(* Logix 5000 AddOnInstructionDefinition export Banner_DFG1_Param_v4; software revision 32.00 *)

TYPE Banner_DFG1_RD_v2 :   // UDT with all of the Read only parameters for DFG1.
STRUCT
   Master_Cycle_Time : INT;
   Min_Cycle_Time : INT;
   M_Sequence_Capability : INT;
   IO_Link_Version_ID : INT;
   Process_Data_Input_Length : INT;
   Process_Data_Output_Length : INT;
   Combined_Vendor_ID : DINT;   // IO-Link Vendor ID
   Vendor_ID1 : INT;
   Vendor_ID2 : INT;
   Combined_Device_ID : DINT;   // IO-Link Device ID
   Device_ID1 : INT;
   Device_ID2 : INT;
   Device_ID3 : INT;
   Serial_Number : STRING;
   Teach_State : SINT;   // 0 =IDLE, 1 = SP1 Success, 4 = Wait for Command, 5 = Busy, 7 = Error
   SP1_TP1 : SINT;   // 0 = Teach point 1 not taught or not successful, 1 = Teach point 1 was successful
   SP1_TP2 : SINT;   // 0 = Teach point 2 not taught or not successful, 1 = Teach point 2 was successful
   SP2_TP1 : SINT;   // 0 = Teach point 2 not taught or not successful, 1 = Teach point 2 was successful
   SP2_TP2 : SINT;   // 0 = Teach point 2 not taught or not successful, 1 = Teach point 2 was successful
   Output_Mode : SINT;   // 0 = Dark Operate, 1 = Light Operate.
   Lower_Hysteresis : DINT;
   Lower_Threshold : DINT;
   Reference : DINT;
   Upper_Hysteresis : DINT;
   Upper_Threshold : DINT;
   Max_Adjustable_Reference : DINT;
   Min_Adjustable_Reference : DINT;
   Max_Teachable_Reference : DINT;
   Min_Teachable_Reference : DINT;
END_STRUCT
END_TYPE

TYPE Banner_DFG1_v2 :   // UDT with all of the parameters needed to work with a Banner DF-G1 IO-Link Sensor.
STRUCT
   Initial_Global_Read : BOOL;   // Determines if all of the IO-Link data has been read into the PLC yet
   Command : INT;   // Value placed in here will activate a read or write to a specifc IO-Link Index
   Read_Data : Banner_DFG1_RD_v2;
   Write_Data : Banner_DFG1_WD_v2;
   Archive_Data : Banner_DFG1_WD_v2;
   Reset : BOOL;   // Resets AOI. This will force a complete parameter read of the sensor.
END_STRUCT
END_TYPE

TYPE Banner_DFG1_WD_v2 :   // UDT with all of the Write only parameters for DFG1.
STRUCT
   System_Command : INT;   // See IODD file for list of commands that can be activated via the System Command interface
   Parameter_Access_Lock : SINT;   // Write access to all read/write parameters is block when this bit is ON.
   Data_Storage_Lock : SINT;   // Data storage mechanism is inhibited when bit is ON.
   Local_Parameterization_Lock : SINT;   // Parameteriation via local control elementes is inhibited.
   Local_User_Interface_Lock : SINT;   // Operation of the hmi on the device is disabled.
   BDC1_Setpoint_SP1 : DINT;   // Switch point value
   BDC1_Setpoint_SP2 : DINT;   // Unused
   BDC1_Swithpoint_Logic : INT;   // 0 = Light Operate, 1 = Dark Operate
   BDC1_BDC_Mode : INT;   // 1 = Single Point, 128 = Window Set, 129 = Light Set, 130 = Dark Set
   BDC1_Hysteresis : DINT;   // User selectable Hysteresis. 0 = 1.0x, 1 = 1.5x, and 2 = 2.5x.
   Off_Delay_On_Oneshot_Time : DINT;   // Delay in ms.
   On_Delay_Off_Oneshot_Time : DINT;   // Delay in ms.
   Delay_Mode : SINT;   // 0 = Off On Delay, 3 = Off Oneshot, 12 = On Oneshot.
   Process_Data_Filter_Update_Time : DINT;   // Value*.1ms. Amount of time to collect average sample for process data.
   Auto_Threshold_Response_Time : INT;   // 14 = 2.5s, 15 = 5s, 16 = 10s, 17 = 20s. Used in Light/Dark/Window Set only.
   Offset_Percent : DINT;   // Offset percent from taught condition in Window, Light or Dark Set modes only.
   Auto_Treshold : SINT;   // 0 = Disabled, 3 = Enabled. Algorithm caontinuously tracks slow changes in taught condition and optimizes thresholds.
   Teach_Selection : INT;   // 0 = 2Pt, 1 = Dynamic, 2 = Window, 3 = Light, 4 = Dark, 5 = Cal.
   Response_Speed : INT;   // 0 = 200, 1 = 500, 2 = 2000, 3 = 5000 microseconds.
   Gain_Mode : SINT;   // 0 = Fixed, 2 = Auto.
   Gain_Level : SINT;   // 0 = Gain 1, 1 = Gain 2, 2 = Gain 3, 3 = Gain 4, 4= Gain 5, 5 = Gain 6, 6 = Gain 7, 7 = Gain 8.
   Display_Orientation : SINT;   // 0 = Normal, 1 = Flipped.
   ECO_Mode : SINT;   // 0 = Disabled, 1 = Enabled.
   Signal_Theshold_Readout : SINT;   // 0 = Numeric, 1 = Percentage.
END_STRUCT
END_TYPE

TYPE Banner_IOL_Port_v4 :   // UDT that has all of the data items necessary to communicate with a specific Port on a IO-Link Master
STRUCT
   Port_Controlled : INT;   // Each bit represents a port on an IO-Link Master. Set to 1 to tell AOI to control that port.
   Port_Activate : INT;   // Each bit represents a port on an IO-Link Master. When ON that port will process any commands in queue.
   Port_Read : INT;   // Each bit represents a port on an IO-Link Master. Used to determine when device AOI has requested a Read command.
   Port_Write : INT;   // Each bit represents a port on an IO-Link Master. Used to determine when device AOI has requested a Write command.
   Port_RW_Complete : INT;   // Each bit represents a port on an IO-Link Master. Tells device AOI that Read or Write request has been completed.
   Port_Device_Read : INT;
   Data_Transfer : SINT[190];   // Array to transfer data from IO-Master to device AOIs.
END_STRUCT
END_TYPE

ADD_ON_INSTRUCTION Banner_DFG1_Param_v4   (* revision 4.0, vendor Banner Engineering *)
// AOI to read and write parameter data to an IO-Link DF-G1.
VAR_IN_OUT
   DFG1 : Banner_DFG1_v2; {required}
   Port_Data : Banner_IOL_Port_v4; {required}
END_VAR
VAR_INPUT
   Port : DINT; {required}
END_VAR
VAR
   Local_Control : DINT; {access None}
   Global_Read_Command_Value : INT; {access None}
   Global_Write_Command_Value : INT; {access None}
   Error_Generated : BOOL; {access None}
   Command_Being_Processed : BOOL; {access None}
   Update_Archive : BOOL; {access None}
   Index_Write_Inprocess : DINT; {access None}
   Index_Write_Control : DINT; {access None}
   Inprocess_Index : DINT; {access None}
END_VAR

ROUTINE Logic   (* ladder *)
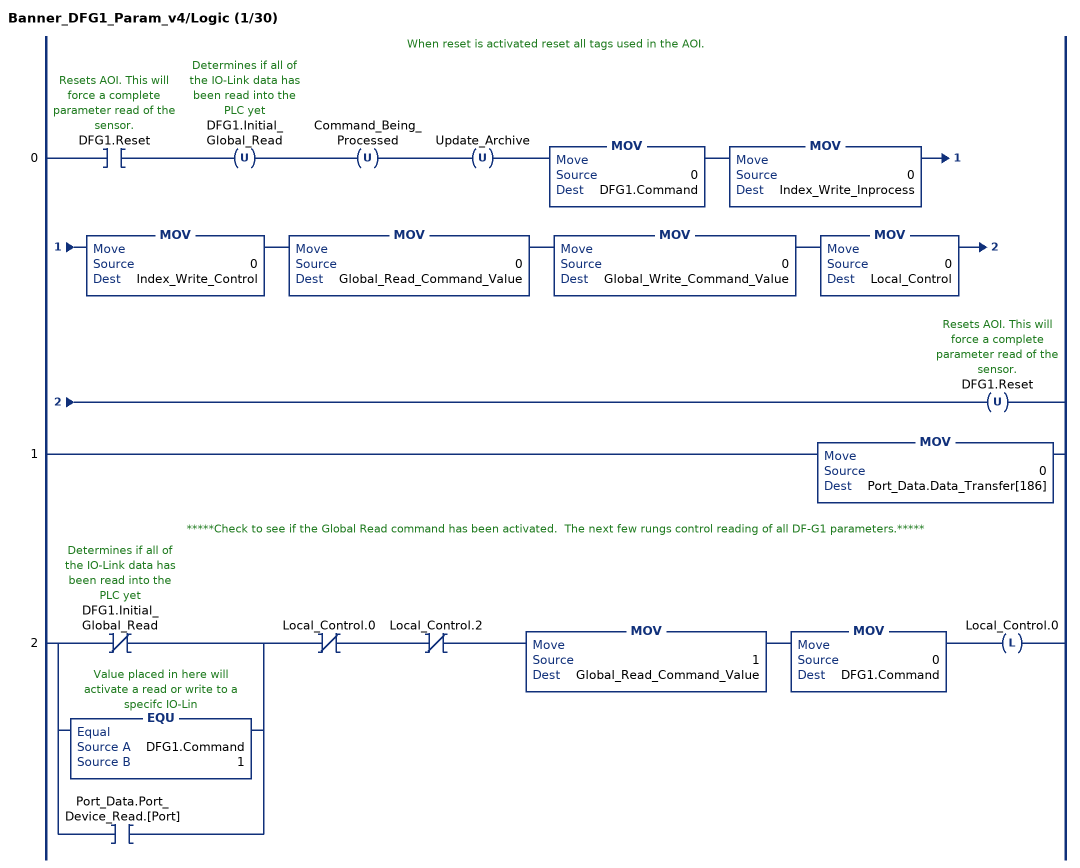
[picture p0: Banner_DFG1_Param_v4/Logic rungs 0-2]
   // When reset is activated reset all tags used in the AOI.
   0: XIC(DFG1.Reset)OTU(DFG1.Initial_Global_Read)OTU(Command_Being_Processed)OTU(Update_Archive)MOV(0,DFG1.Command)MOV(0,Index_Write_Inprocess)MOV(0,Index_Write_Control)MOV(0,Global_Read_Command_Value)MOV(0,Global_Write_Command_Value)MOV(0,Local_Control)OTU(DFG1.Reset);
   1: MOV(0,Port_Data.Data_Transfer[186]);
   // *****Check to see if the Global Read command has been activated.  The next few rungs control reading of all DF-G1 parameters.*****
   2: [XIO(DFG1.Initial_Global_Read) ,EQU(DFG1.Command,1) ,XIC(Port_Data.Port_Device_Read.[Port]) ]XIO(Local_Control.0)XIO(Local_Control.2)MOV(1,Global_Read_Command_Value)MOV(0,DFG1.Command)OTL(Local_Control.0);
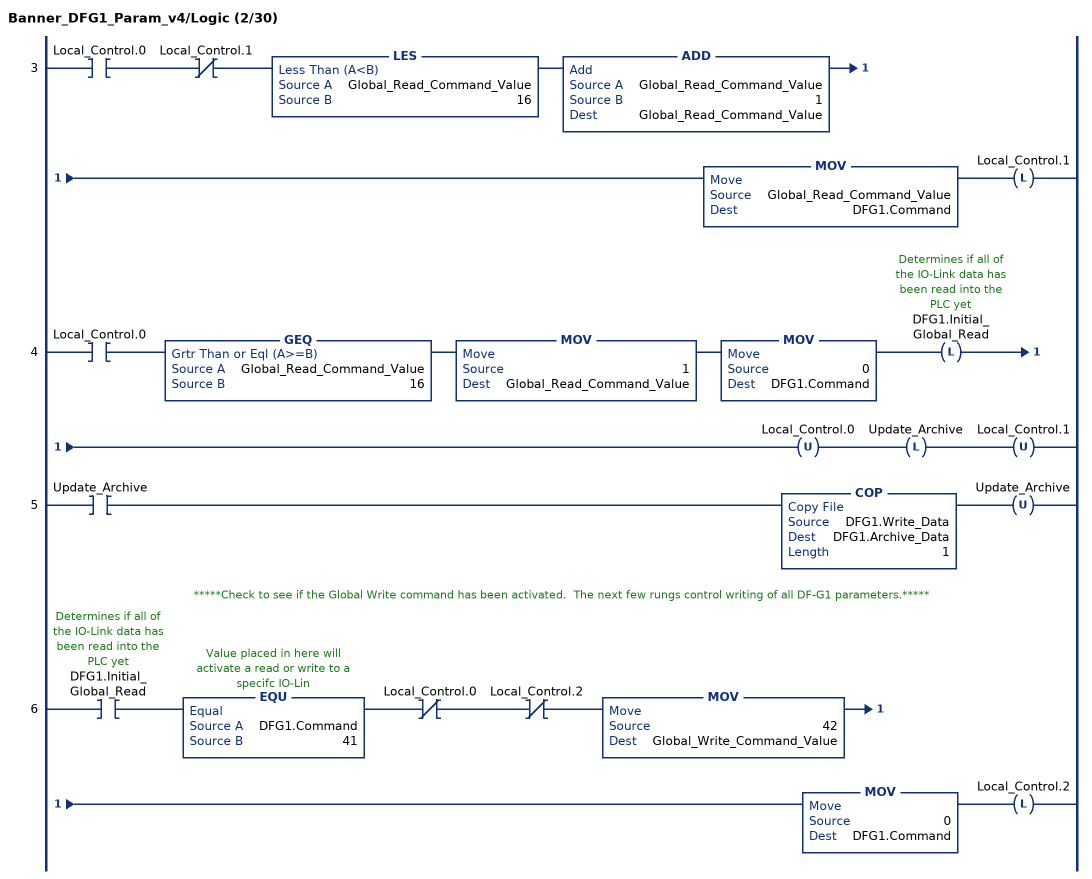
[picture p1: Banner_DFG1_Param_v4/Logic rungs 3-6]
   3: XIC(Local_Control.0)XIO(Local_Control.1)LES(Global_Read_Command_Value,16)ADD(Global_Read_Command_Value,1,Global_Read_Command_Value)MOV(Global_Read_Command_Value,DFG1.Command)OTL(Local_Control.1);
   4: XIC(Local_Control.0)GEQ(Global_Read_Command_Value,16)MOV(1,Global_Read_Command_Value)MOV(0,DFG1.Command)OTL(DFG1.Initial_Global_Read)OTU(Local_Control.0)OTL(Update_Archive)OTU(Local_Control.1);
   5: XIC(Update_Archive)COP(DFG1.Write_Data,DFG1.Archive_Data,1)OTU(Update_Archive);
   // *****Check to see if the Global Write command has been activated.  The next few rungs control writing of all DF-G1 parameters.*****
   6: XIC(DFG1.Initial_Global_Read)EQU(DFG1.Command,41)XIO(Local_Control.0)XIO(Local_Control.2)MOV(42,Global_Write_Command_Value)MOV(0,DFG1.Command)OTL(Local_Control.2);
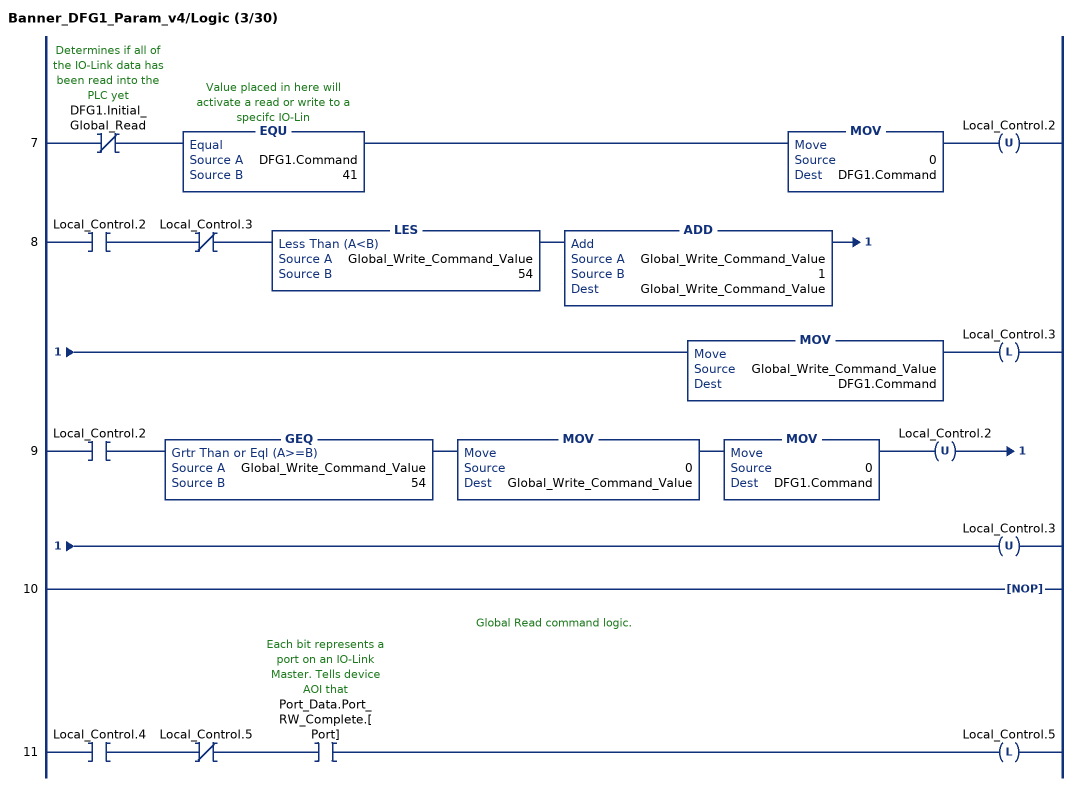
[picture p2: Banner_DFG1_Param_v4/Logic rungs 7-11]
   7: XIO(DFG1.Initial_Global_Read)EQU(DFG1.Command,41)MOV(0,DFG1.Command)OTU(Local_Control.2);
   8: XIC(Local_Control.2)XIO(Local_Control.3)LES(Global_Write_Command_Value,54)ADD(Global_Write_Command_Value,1,Global_Write_Command_Value)MOV(Global_Write_Command_Value,DFG1.Command)OTL(Local_Control.3);
   9: XIC(Local_Control.2)GEQ(Global_Write_Command_Value,54)MOV(0,Global_Write_Command_Value)MOV(0,DFG1.Command)OTU(Local_Control.2)OTU(Local_Control.3);
   10: NOP();
   // Global Read command logic.
   11: XIC(Local_Control.4)XIO(Local_Control.5)XIC(Port_Data.Port_RW_Complete.[Port])OTL(Local_Control.5);
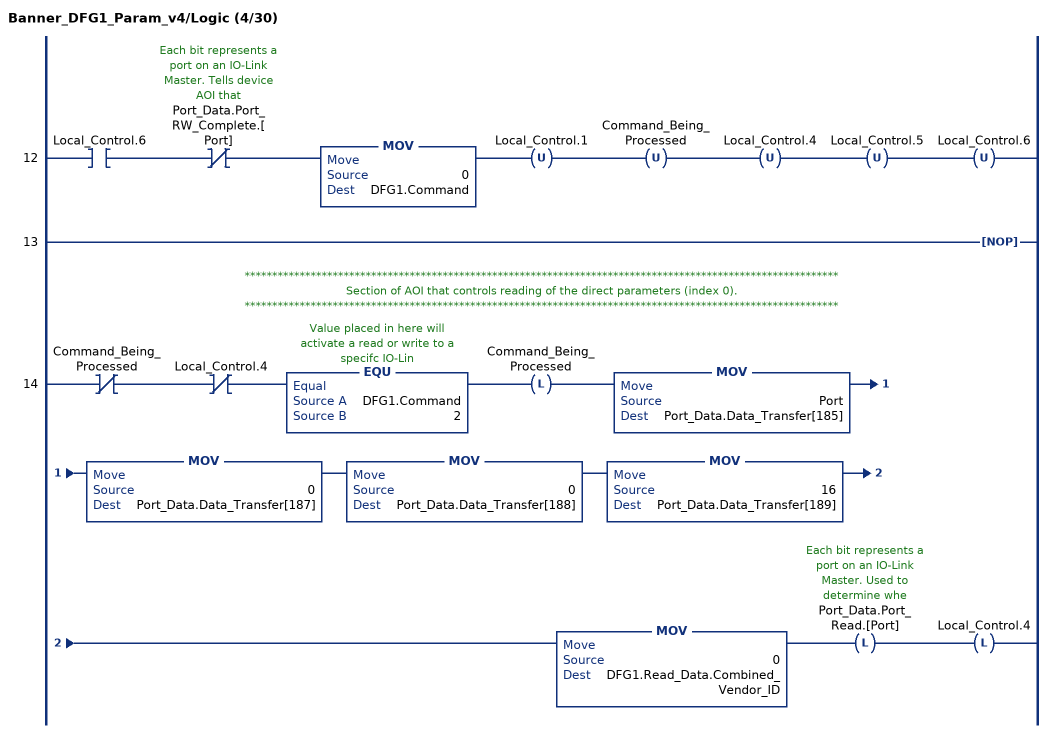
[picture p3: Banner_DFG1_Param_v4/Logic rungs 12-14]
   12: XIC(Local_Control.6)XIO(Port_Data.Port_RW_Complete.[Port])MOV(0,DFG1.Command)OTU(Local_Control.1)OTU(Command_Being_Processed)OTU(Local_Control.4)OTU(Local_Control.5)OTU(Local_Control.6);
   13: NOP();
   // ************************************************************************************************************
   // Section of AOI that controls reading of the direct parameters (index 0).
   // ************************************************************************************************************
   14: XIO(Command_Being_Processed)XIO(Local_Control.4)EQU(DFG1.Command,2)OTL(Command_Being_Processed)MOV(Port,Port_Data.Data_Transfer[185])MOV(0,Port_Data.Data_Transfer[187])MOV(0,Port_Data.Data_Transfer[188])MOV(16,Port_Data.Data_Transfer[189])MOV(0,DFG1.Read_Data.Combined_Vendor_ID)OTL(Port_Data.Port_Read.[Port])OTL(Local_Control.4);
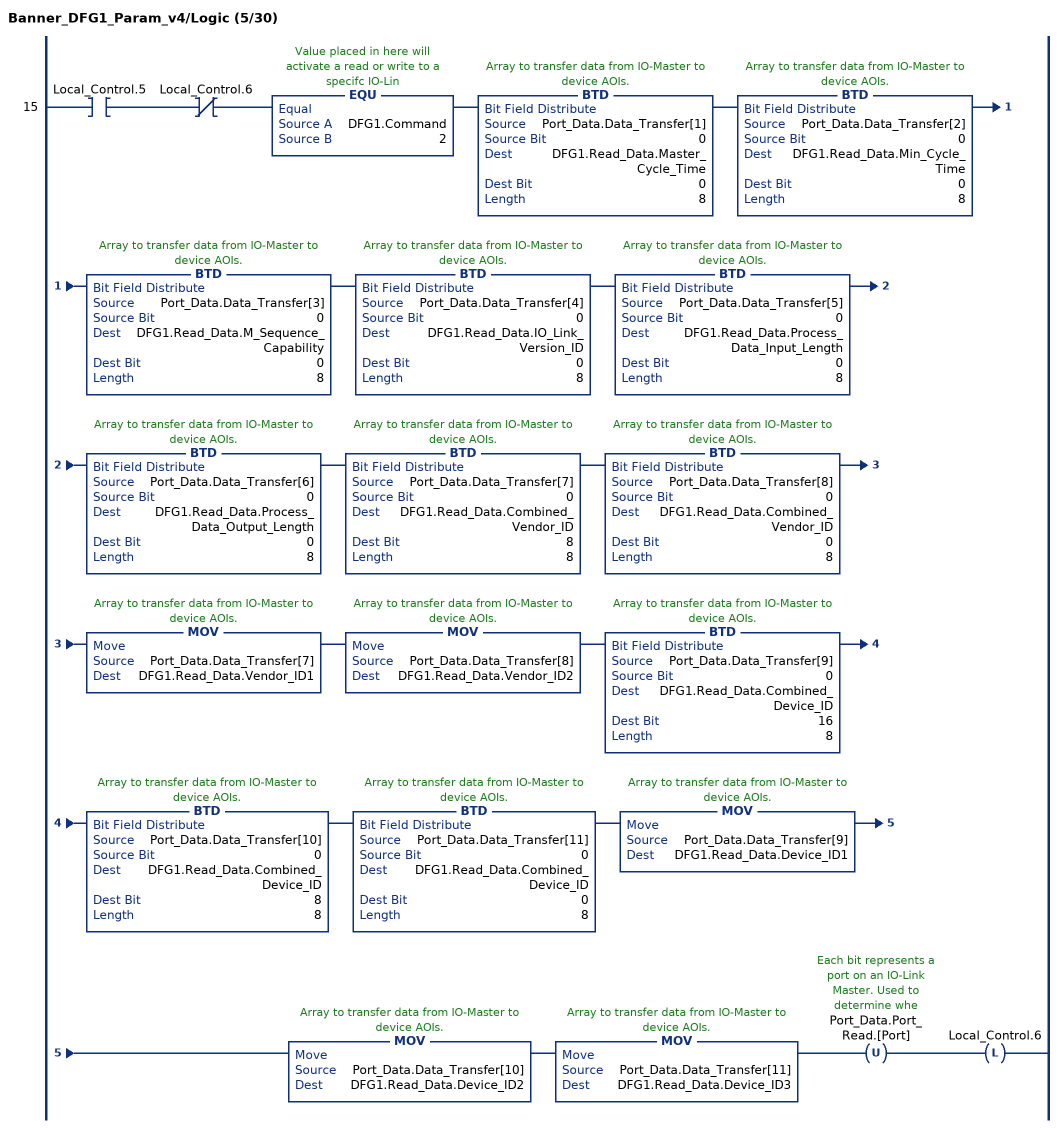
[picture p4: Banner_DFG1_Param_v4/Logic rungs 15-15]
   15: XIC(Local_Control.5)XIO(Local_Control.6)EQU(DFG1.Command,2)BTD(Port_Data.Data_Transfer[1],0,DFG1.Read_Data.Master_Cycle_Time,0,8)BTD(Port_Data.Data_Transfer[2],0,DFG1.Read_Data.Min_Cycle_Time,0,8)BTD(Port_Data.Data_Transfer[3],0,DFG1.Read_Data.M_Sequence_Capability,0,8)BTD(Port_Data.Data_Transfer[4],0,DFG1.Read_Data.IO_Link_Version_ID,0,8)BTD(Port_Data.Data_Transfer[5],0,DFG1.Read_Data.Process_Data_Input_Length,0,8)BTD(Port_Data.Data_Transfer[6],0,DFG1.Read_Data.Process_Data_Output_Length,0,8)BTD(Port_Data.Data_Transfer[7],0,DFG1.Read_Data.Combined_Vendor_ID,8,8)BTD(Port_Data.Data_Transfer[8],0,DFG1.Read_Data.Combined_Vendor_ID,0,8)MOV(Port_Data.Data_Transfer[7],DFG1.Read_Data.Vendor_ID1)MOV(Port_Data.Data_Transfer[8],DFG1.Read_Data.Vendor_ID2)BTD(Port_Data.Data_Transfer[9],0,DFG1.Read_Data.Combined_Device_ID,16,8)BTD(Port_Data.Data_Transfer[10],0,DFG1.Read_Data.Combined_Device_ID,8,8)BTD(Port_Data.Data_Transfer[11],0,DFG1.Read_Data.Combined_Device_ID,0,8)MOV(Port_Data.Data_Transfer[9],DFG1.Read_Data.Device_ID1)MOV(Port_Data.Data_Transfer[10],DFG1.Read_Data.Device_ID2)MOV(Port_Data.Data_Transfer[11],DFG1.Read_Data.Device_ID3)OTU(Port_Data.Port_Read.[Port])OTL(Local_Control.6);
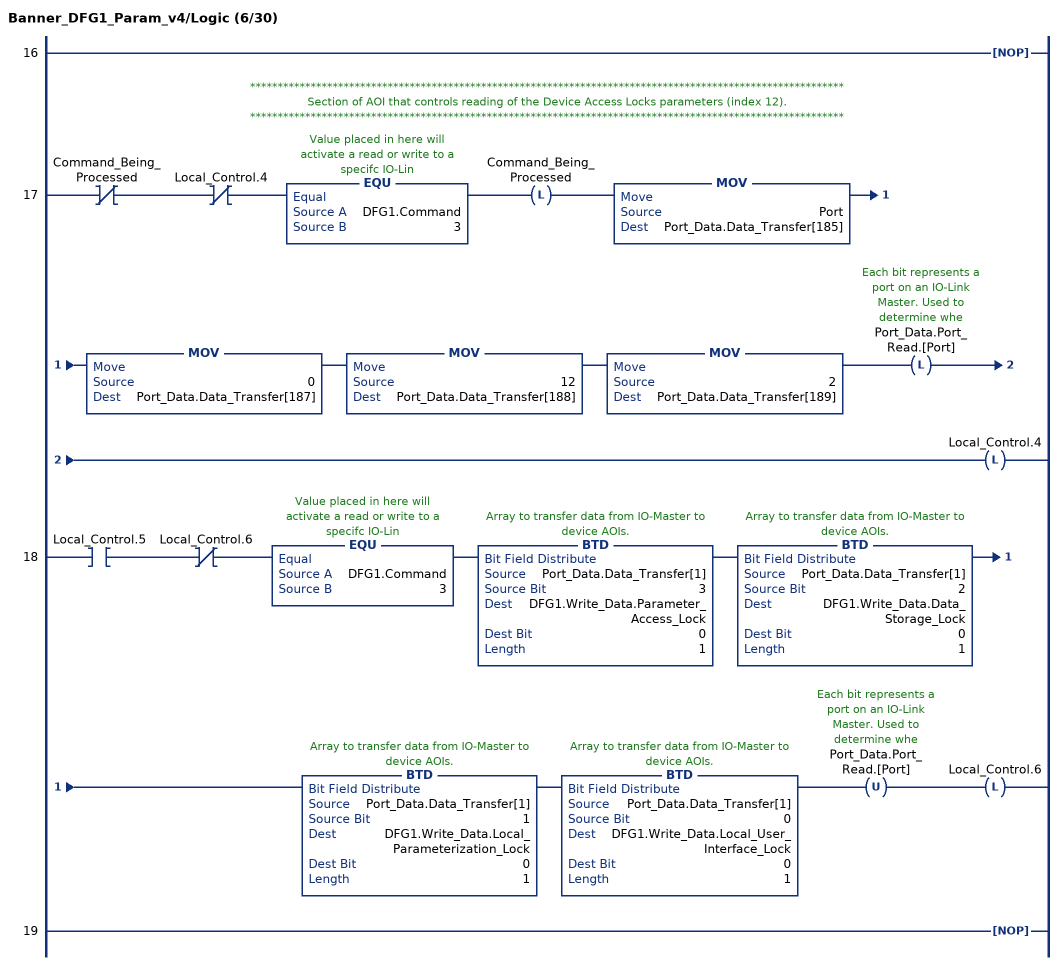
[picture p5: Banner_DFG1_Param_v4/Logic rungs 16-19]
   16: NOP();
   // ************************************************************************************************************
   // Section of AOI that controls reading of the Device Access Locks parameters (index 12).
   // ************************************************************************************************************
   17: XIO(Command_Being_Processed)XIO(Local_Control.4)EQU(DFG1.Command,3)OTL(Command_Being_Processed)MOV(Port,Port_Data.Data_Transfer[185])MOV(0,Port_Data.Data_Transfer[187])MOV(12,Port_Data.Data_Transfer[188])MOV(2,Port_Data.Data_Transfer[189])OTL(Port_Data.Port_Read.[Port])OTL(Local_Control.4);
   18: XIC(Local_Control.5)XIO(Local_Control.6)EQU(DFG1.Command,3)BTD(Port_Data.Data_Transfer[1],3,DFG1.Write_Data.Parameter_Access_Lock,0,1)BTD(Port_Data.Data_Transfer[1],2,DFG1.Write_Data.Data_Storage_Lock,0,1)BTD(Port_Data.Data_Transfer[1],1,DFG1.Write_Data.Local_Parameterization_Lock,0,1)BTD(Port_Data.Data_Transfer[1],0,DFG1.Write_Data.Local_User_Interface_Lock,0,1)OTU(Port_Data.Port_Read.[Port])OTL(Local_Control.6);
   19: NOP();
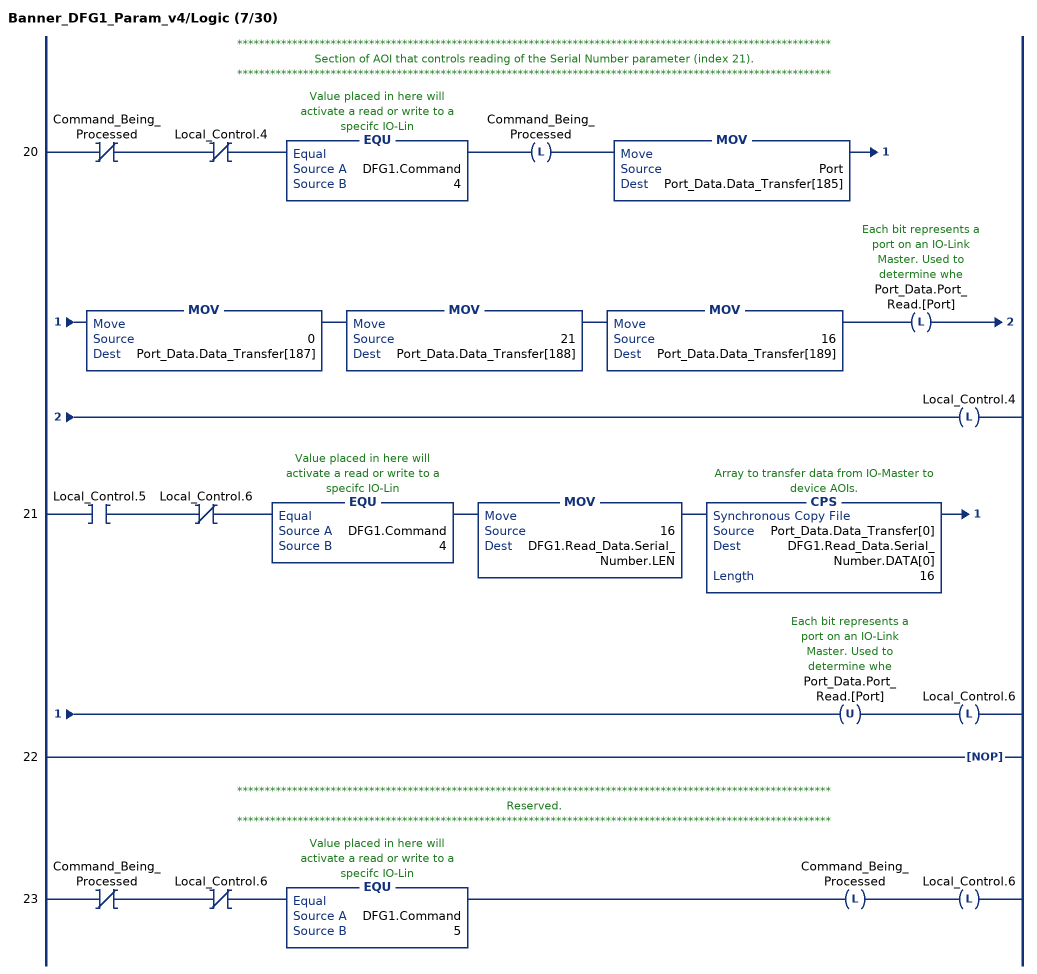
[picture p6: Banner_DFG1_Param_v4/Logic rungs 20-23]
   // ************************************************************************************************************
   // Section of AOI that controls reading of the Serial Number parameter (index 21).
   // ************************************************************************************************************
   20: XIO(Command_Being_Processed)XIO(Local_Control.4)EQU(DFG1.Command,4)OTL(Command_Being_Processed)MOV(Port,Port_Data.Data_Transfer[185])MOV(0,Port_Data.Data_Transfer[187])MOV(21,Port_Data.Data_Transfer[188])MOV(16,Port_Data.Data_Transfer[189])OTL(Port_Data.Port_Read.[Port])OTL(Local_Control.4);
   21: XIC(Local_Control.5)XIO(Local_Control.6)EQU(DFG1.Command,4)MOV(16,DFG1.Read_Data.Serial_Number.LEN)CPS(Port_Data.Data_Transfer[0],DFG1.Read_Data.Serial_Number.DATA[0],16)OTU(Port_Data.Port_Read.[Port])OTL(Local_Control.6);
   22: NOP();
   // ************************************************************************************************************
   // Reserved.
   // ************************************************************************************************************
   23: XIO(Command_Being_Processed)XIO(Local_Control.6)EQU(DFG1.Command,5)OTL(Command_Being_Processed)OTL(Local_Control.6);
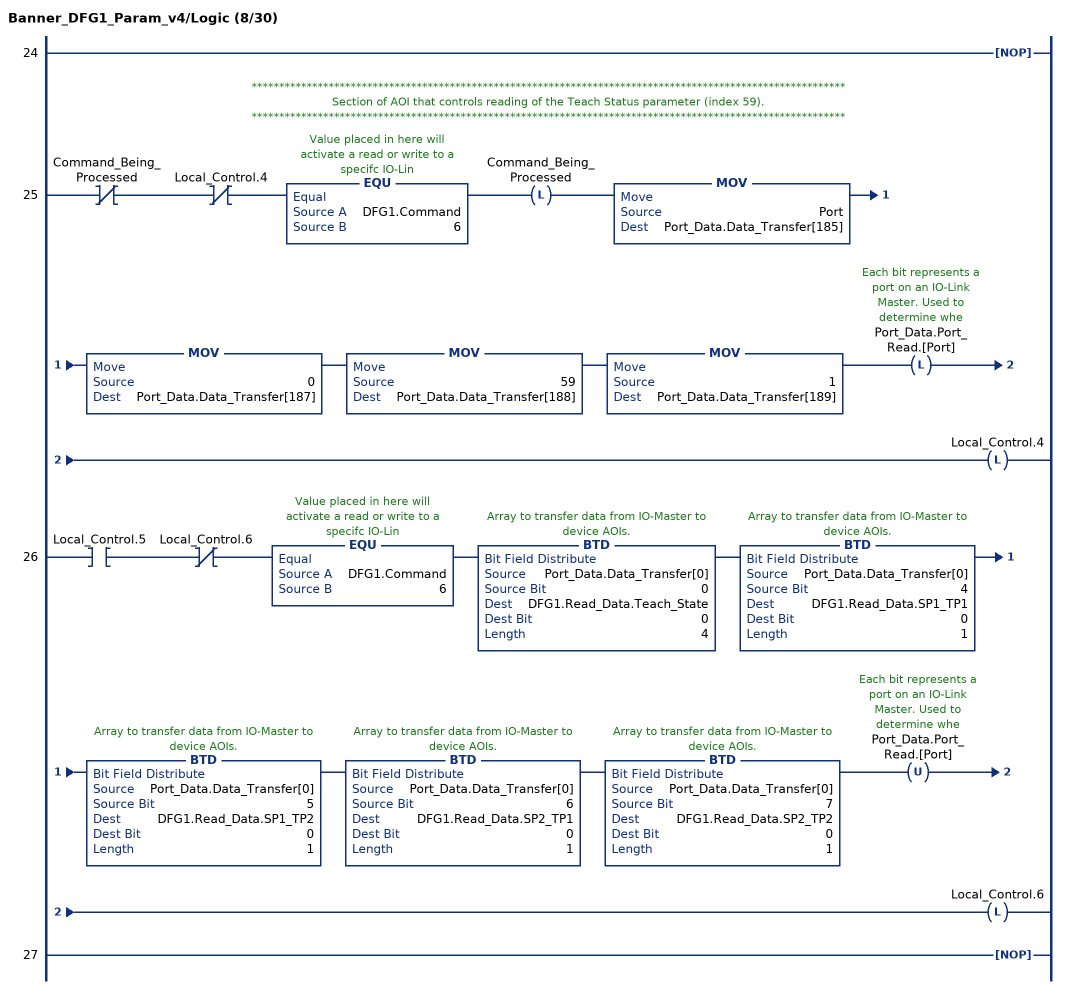
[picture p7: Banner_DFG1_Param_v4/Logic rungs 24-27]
   24: NOP();
   // ************************************************************************************************************
   // Section of AOI that controls reading of the Teach Status parameter (index 59).
   // ************************************************************************************************************
   25: XIO(Command_Being_Processed)XIO(Local_Control.4)EQU(DFG1.Command,6)OTL(Command_Being_Processed)MOV(Port,Port_Data.Data_Transfer[185])MOV(0,Port_Data.Data_Transfer[187])MOV(59,Port_Data.Data_Transfer[188])MOV(1,Port_Data.Data_Transfer[189])OTL(Port_Data.Port_Read.[Port])OTL(Local_Control.4);
   26: XIC(Local_Control.5)XIO(Local_Control.6)EQU(DFG1.Command,6)BTD(Port_Data.Data_Transfer[0],0,DFG1.Read_Data.Teach_State,0,4)BTD(Port_Data.Data_Transfer[0],4,DFG1.Read_Data.SP1_TP1,0,1)BTD(Port_Data.Data_Transfer[0],5,DFG1.Read_Data.SP1_TP2,0,1)BTD(Port_Data.Data_Transfer[0],6,DFG1.Read_Data.SP2_TP1,0,1)BTD(Port_Data.Data_Transfer[0],7,DFG1.Read_Data.SP2_TP2,0,1)OTU(Port_Data.Port_Read.[Port])OTL(Local_Control.6);
   27: NOP();
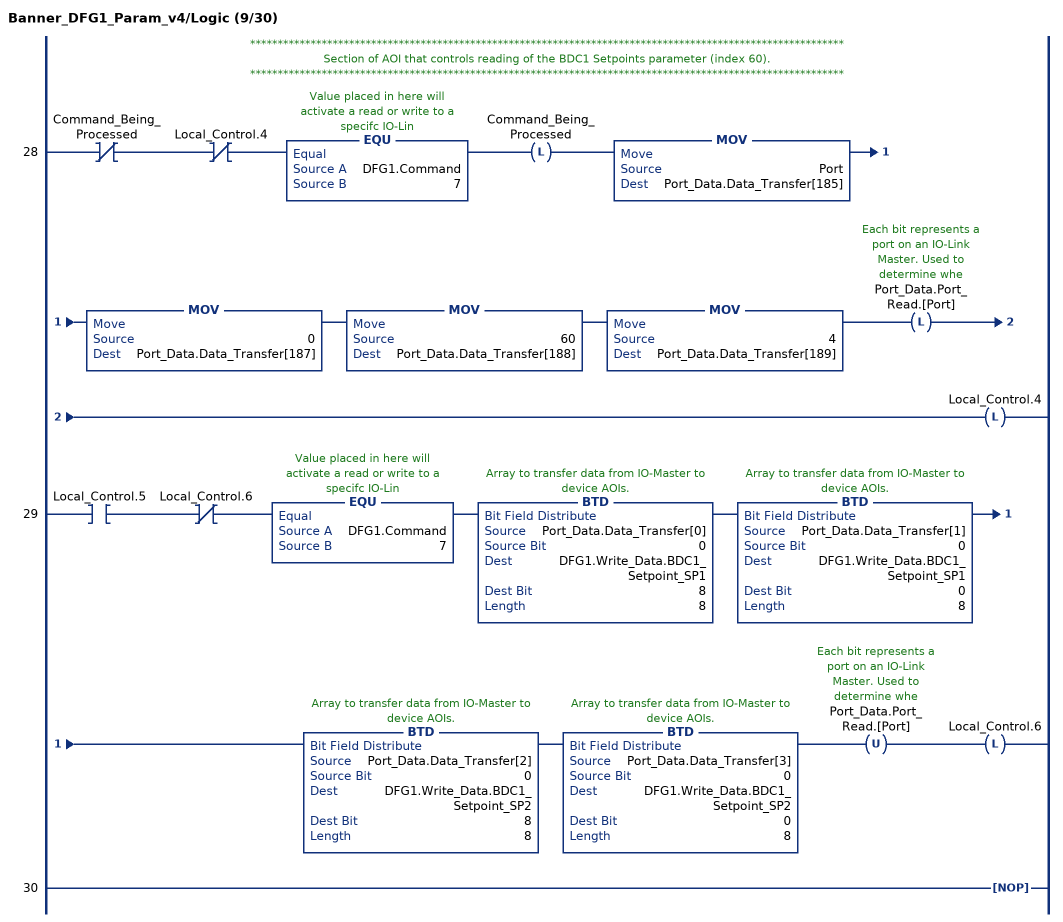
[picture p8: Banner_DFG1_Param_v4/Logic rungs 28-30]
   // ************************************************************************************************************
   // Section of AOI that controls reading of the BDC1 Setpoints parameter (index 60).
   // ************************************************************************************************************
   28: XIO(Command_Being_Processed)XIO(Local_Control.4)EQU(DFG1.Command,7)OTL(Command_Being_Processed)MOV(Port,Port_Data.Data_Transfer[185])MOV(0,Port_Data.Data_Transfer[187])MOV(60,Port_Data.Data_Transfer[188])MOV(4,Port_Data.Data_Transfer[189])OTL(Port_Data.Port_Read.[Port])OTL(Local_Control.4);
   29: XIC(Local_Control.5)XIO(Local_Control.6)EQU(DFG1.Command,7)BTD(Port_Data.Data_Transfer[0],0,DFG1.Write_Data.BDC1_Setpoint_SP1,8,8)BTD(Port_Data.Data_Transfer[1],0,DFG1.Write_Data.BDC1_Setpoint_SP1,0,8)BTD(Port_Data.Data_Transfer[2],0,DFG1.Write_Data.BDC1_Setpoint_SP2,8,8)BTD(Port_Data.Data_Transfer[3],0,DFG1.Write_Data.BDC1_Setpoint_SP2,0,8)OTU(Port_Data.Port_Read.[Port])OTL(Local_Control.6);
   30: NOP();
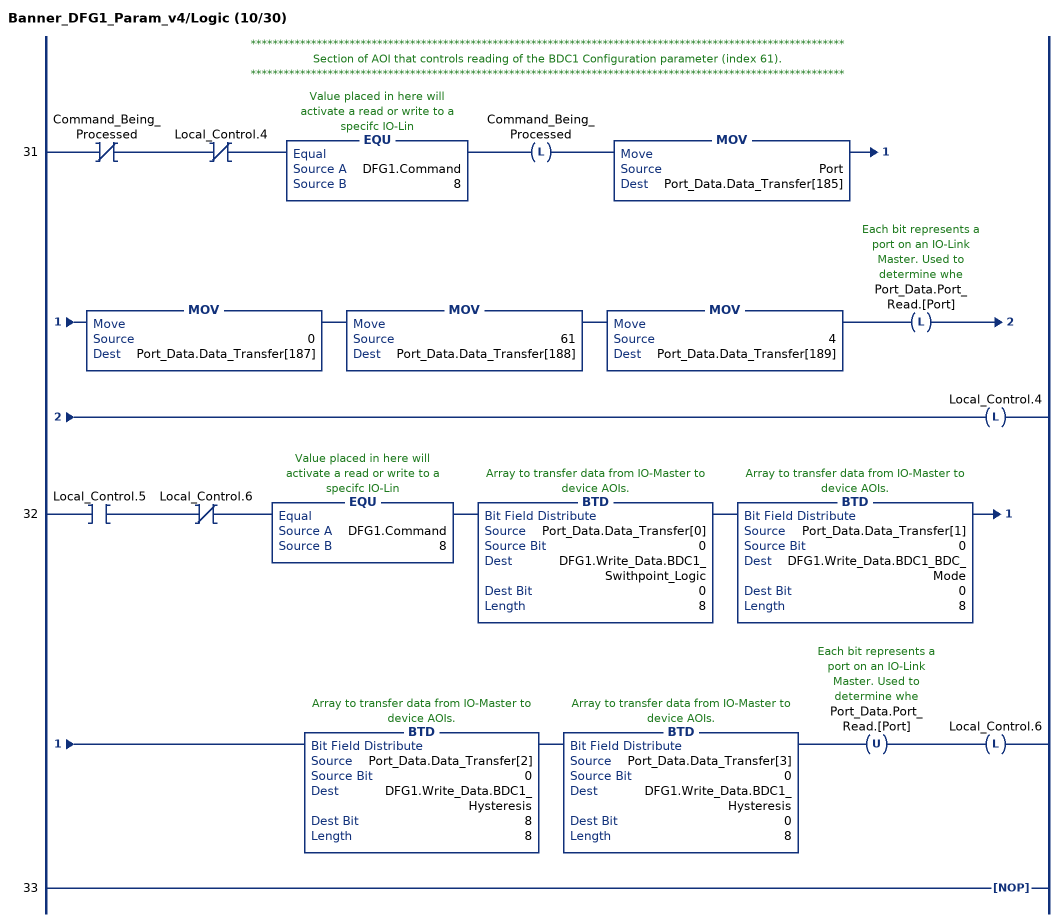
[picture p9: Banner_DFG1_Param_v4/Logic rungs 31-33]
   // ************************************************************************************************************
   // Section of AOI that controls reading of the BDC1 Configuration parameter (index 61).
   // ************************************************************************************************************
   31: XIO(Command_Being_Processed)XIO(Local_Control.4)EQU(DFG1.Command,8)OTL(Command_Being_Processed)MOV(Port,Port_Data.Data_Transfer[185])MOV(0,Port_Data.Data_Transfer[187])MOV(61,Port_Data.Data_Transfer[188])MOV(4,Port_Data.Data_Transfer[189])OTL(Port_Data.Port_Read.[Port])OTL(Local_Control.4);
   32: XIC(Local_Control.5)XIO(Local_Control.6)EQU(DFG1.Command,8)BTD(Port_Data.Data_Transfer[0],0,DFG1.Write_Data.BDC1_Swithpoint_Logic,0,8)BTD(Port_Data.Data_Transfer[1],0,DFG1.Write_Data.BDC1_BDC_Mode,0,8)BTD(Port_Data.Data_Transfer[2],0,DFG1.Write_Data.BDC1_Hysteresis,8,8)BTD(Port_Data.Data_Transfer[3],0,DFG1.Write_Data.BDC1_Hysteresis,0,8)OTU(Port_Data.Port_Read.[Port])OTL(Local_Control.6);
   33: NOP();
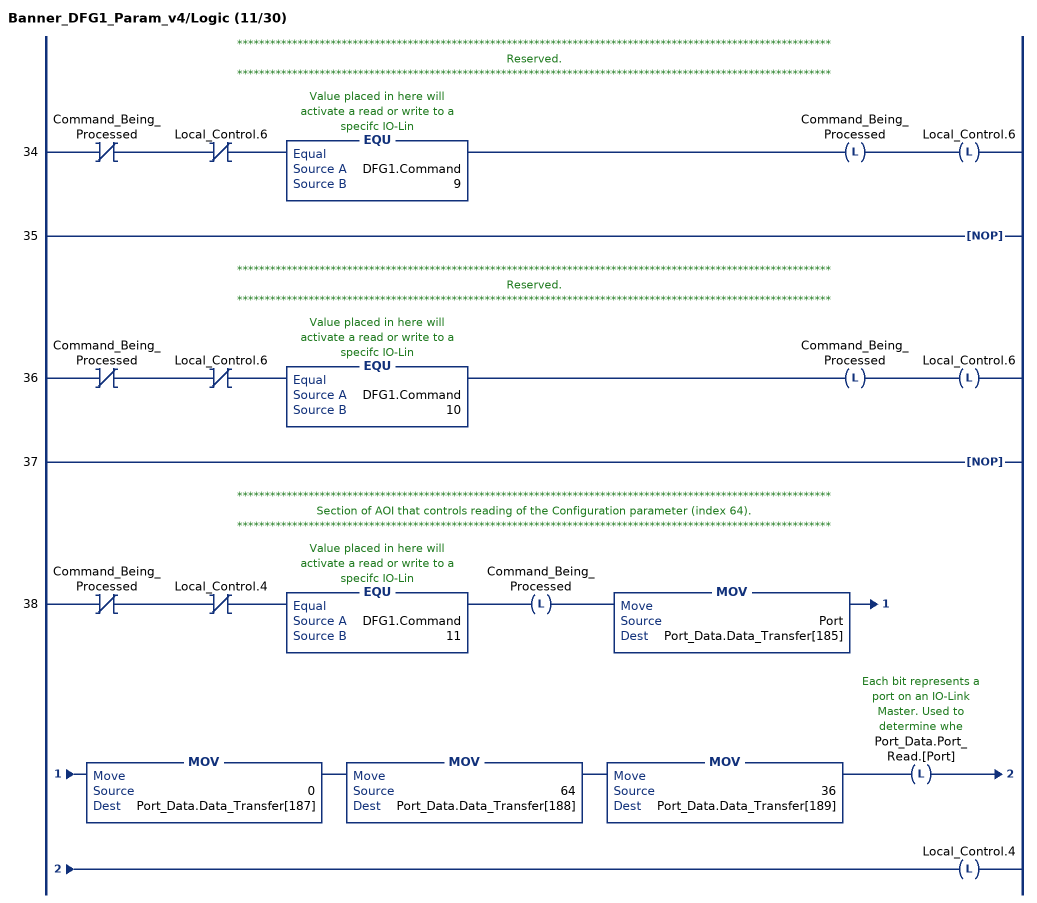
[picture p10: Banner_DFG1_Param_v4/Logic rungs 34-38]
   // ************************************************************************************************************
   // Reserved.
   // ************************************************************************************************************
   34: XIO(Command_Being_Processed)XIO(Local_Control.6)EQU(DFG1.Command,9)OTL(Command_Being_Processed)OTL(Local_Control.6);
   35: NOP();
   // ************************************************************************************************************
   // Reserved.
   // ************************************************************************************************************
   36: XIO(Command_Being_Processed)XIO(Local_Control.6)EQU(DFG1.Command,10)OTL(Command_Being_Processed)OTL(Local_Control.6);
   37: NOP();
   // ************************************************************************************************************
   // Section of AOI that controls reading of the Configuration parameter (index 64).
   // ************************************************************************************************************
   38: XIO(Command_Being_Processed)XIO(Local_Control.4)EQU(DFG1.Command,11)OTL(Command_Being_Processed)MOV(Port,Port_Data.Data_Transfer[185])MOV(0,Port_Data.Data_Transfer[187])MOV(64,Port_Data.Data_Transfer[188])MOV(36,Port_Data.Data_Transfer[189])OTL(Port_Data.Port_Read.[Port])OTL(Local_Control.4);
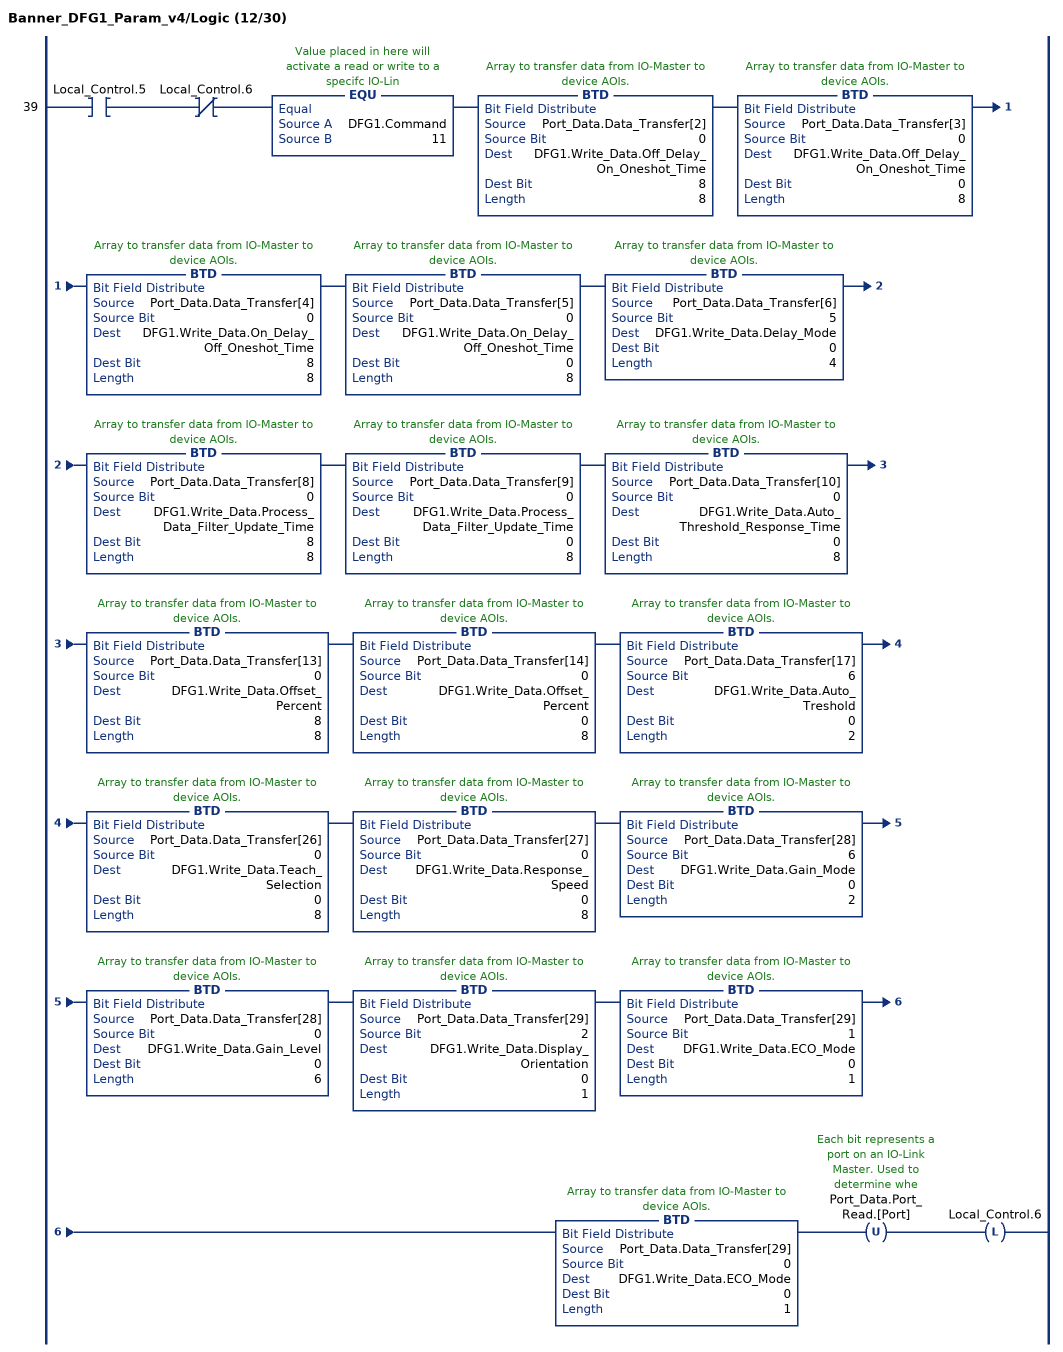
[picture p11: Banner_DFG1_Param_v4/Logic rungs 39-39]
   39: XIC(Local_Control.5)XIO(Local_Control.6)EQU(DFG1.Command,11)BTD(Port_Data.Data_Transfer[2],0,DFG1.Write_Data.Off_Delay_On_Oneshot_Time,8,8)BTD(Port_Data.Data_Transfer[3],0,DFG1.Write_Data.Off_Delay_On_Oneshot_Time,0,8)BTD(Port_Data.Data_Transfer[4],0,DFG1.Write_Data.On_Delay_Off_Oneshot_Time,8,8)BTD(Port_Data.Data_Transfer[5],0,DFG1.Write_Data.On_Delay_Off_Oneshot_Time,0,8)BTD(Port_Data.Data_Transfer[6],5,DFG1.Write_Data.Delay_Mode,0,4)BTD(Port_Data.Data_Transfer[8],0,DFG1.Write_Data.Process_Data_Filter_Update_Time,8,8)BTD(Port_Data.Data_Transfer[9],0,DFG1.Write_Data.Process_Data_Filter_Update_Time,0,8)BTD(Port_Data.Data_Transfer[10],0,DFG1.Write_Data.Auto_Threshold_Response_Time,0,8)BTD(Port_Data.Data_Transfer[13],0,DFG1.Write_Data.Offset_Percent,8,8)BTD(Port_Data.Data_Transfer[14],0,DFG1.Write_Data.Offset_Percent,0,8)BTD(Port_Data.Data_Transfer[17],6,DFG1.Write_Data.Auto_Treshold,0,2)BTD(Port_Data.Data_Transfer[26],0,DFG1.Write_Data.Teach_Selection,0,8)BTD(Port_Data.Data_Transfer[27],0,DFG1.Write_Data.Response_Speed,0,8)BTD(Port_Data.Data_Transfer[28],6,DFG1.Write_Data.Gain_Mode,0,2)BTD(Port_Data.Data_Transfer[28],0,DFG1.Write_Data.Gain_Level,0,6)BTD(Port_Data.Data_Transfer[29],2,DFG1.Write_Data.Display_Orientation,0,1)BTD(Port_Data.Data_Transfer[29],1,DFG1.Write_Data.ECO_Mode,0,1)BTD(Port_Data.Data_Transfer[29],0,DFG1.Write_Data.ECO_Mode,0,1)OTU(Port_Data.Port_Read.[Port])OTL(Local_Control.6);
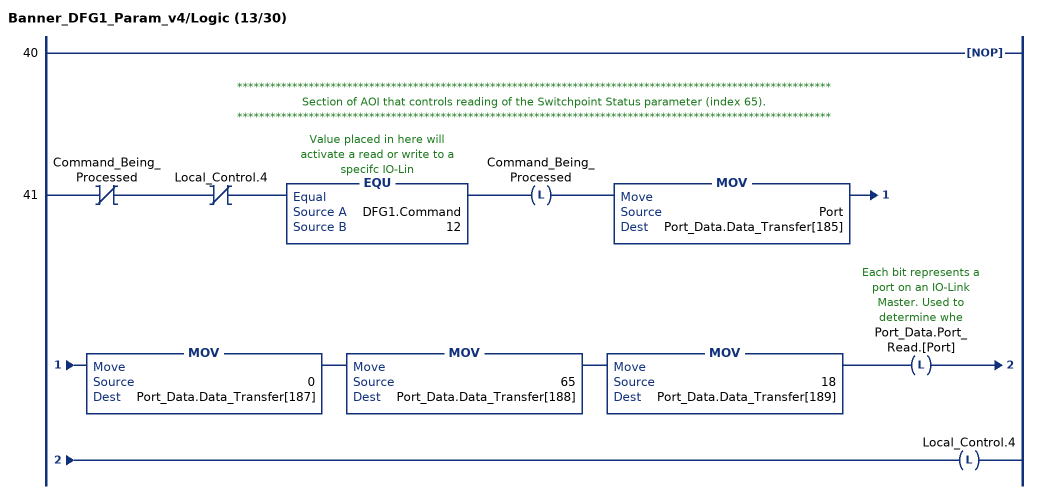
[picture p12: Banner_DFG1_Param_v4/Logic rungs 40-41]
   40: NOP();
   // ************************************************************************************************************
   // Section of AOI that controls reading of the Switchpoint Status parameter (index 65).
   // ************************************************************************************************************
   41: XIO(Command_Being_Processed)XIO(Local_Control.4)EQU(DFG1.Command,12)OTL(Command_Being_Processed)MOV(Port,Port_Data.Data_Transfer[185])MOV(0,Port_Data.Data_Transfer[187])MOV(65,Port_Data.Data_Transfer[188])MOV(18,Port_Data.Data_Transfer[189])OTL(Port_Data.Port_Read.[Port])OTL(Local_Control.4);
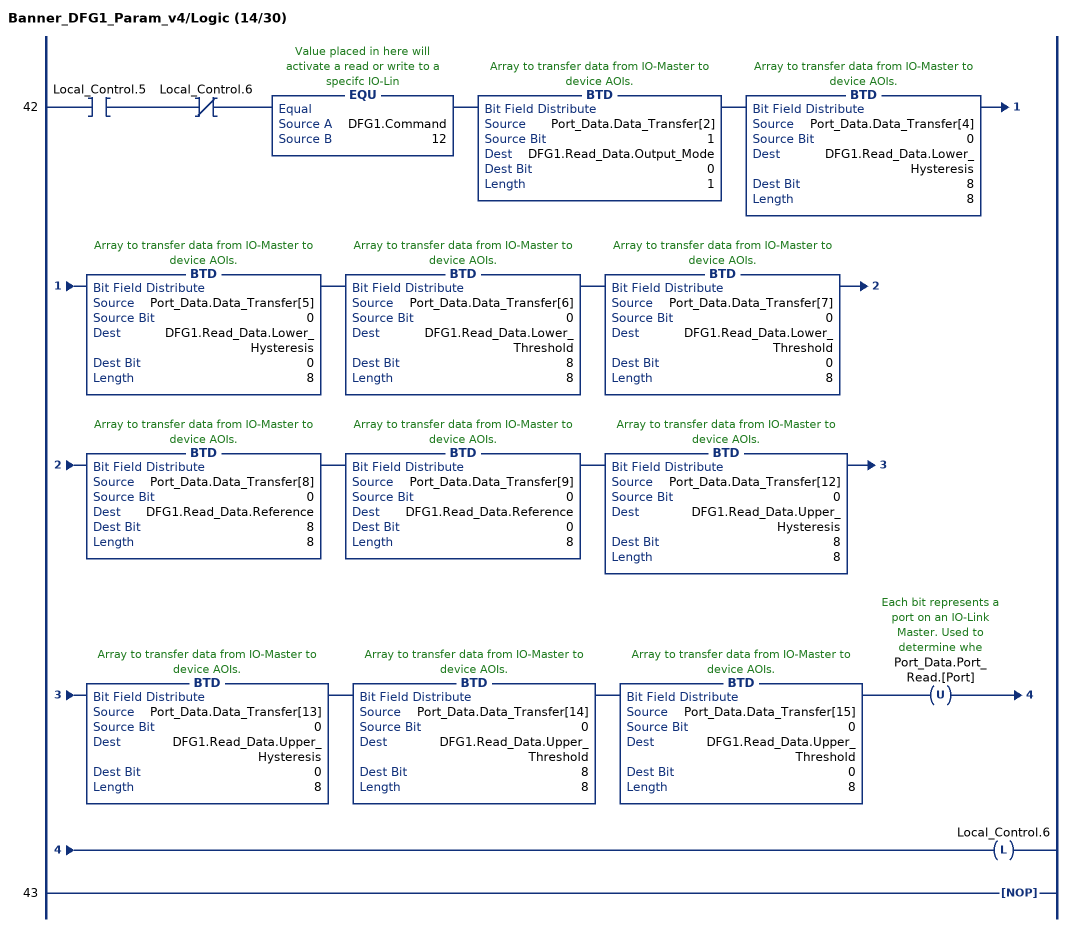
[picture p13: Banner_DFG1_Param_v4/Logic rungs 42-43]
   42: XIC(Local_Control.5)XIO(Local_Control.6)EQU(DFG1.Command,12)BTD(Port_Data.Data_Transfer[2],1,DFG1.Read_Data.Output_Mode,0,1)BTD(Port_Data.Data_Transfer[4],0,DFG1.Read_Data.Lower_Hysteresis,8,8)BTD(Port_Data.Data_Transfer[5],0,DFG1.Read_Data.Lower_Hysteresis,0,8)BTD(Port_Data.Data_Transfer[6],0,DFG1.Read_Data.Lower_Threshold,8,8)BTD(Port_Data.Data_Transfer[7],0,DFG1.Read_Data.Lower_Threshold,0,8)BTD(Port_Data.Data_Transfer[8],0,DFG1.Read_Data.Reference,8,8)BTD(Port_Data.Data_Transfer[9],0,DFG1.Read_Data.Reference,0,8)BTD(Port_Data.Data_Transfer[12],0,DFG1.Read_Data.Upper_Hysteresis,8,8)BTD(Port_Data.Data_Transfer[13],0,DFG1.Read_Data.Upper_Hysteresis,0,8)BTD(Port_Data.Data_Transfer[14],0,DFG1.Read_Data.Upper_Threshold,8,8)BTD(Port_Data.Data_Transfer[15],0,DFG1.Read_Data.Upper_Threshold,0,8)OTU(Port_Data.Port_Read.[Port])OTL(Local_Control.6);
   43: NOP();
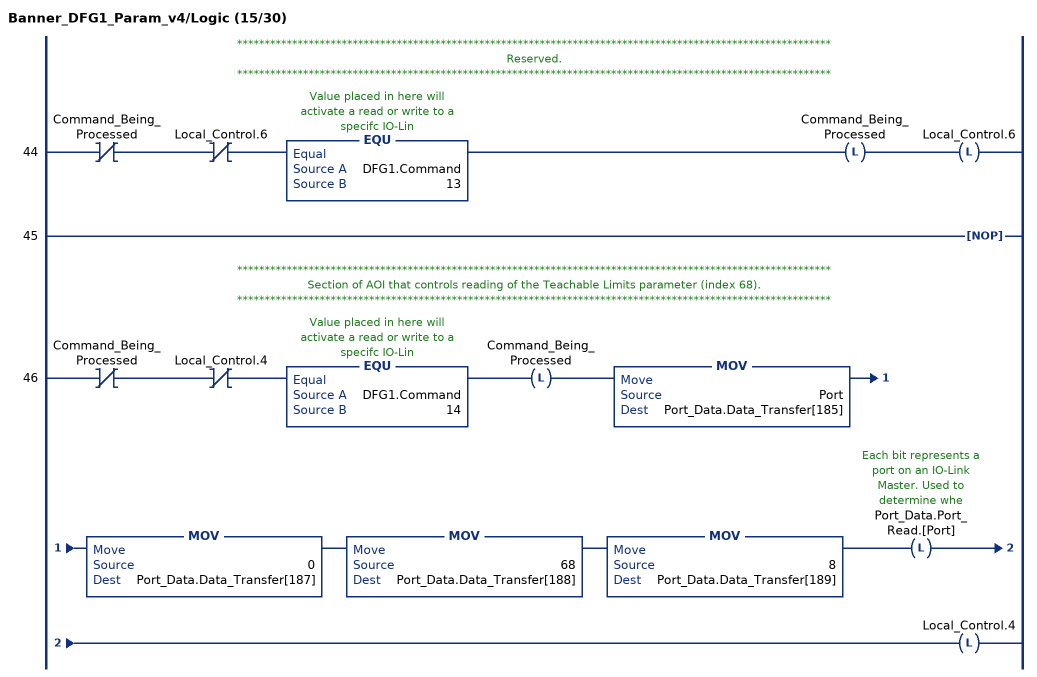
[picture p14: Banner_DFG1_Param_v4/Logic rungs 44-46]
   // ************************************************************************************************************
   // Reserved.
   // ************************************************************************************************************
   44: XIO(Command_Being_Processed)XIO(Local_Control.6)EQU(DFG1.Command,13)OTL(Command_Being_Processed)OTL(Local_Control.6);
   45: NOP();
   // ************************************************************************************************************
   // Section of AOI that controls reading of the Teachable Limits parameter (index 68).
   // ************************************************************************************************************
   46: XIO(Command_Being_Processed)XIO(Local_Control.4)EQU(DFG1.Command,14)OTL(Command_Being_Processed)MOV(Port,Port_Data.Data_Transfer[185])MOV(0,Port_Data.Data_Transfer[187])MOV(68,Port_Data.Data_Transfer[188])MOV(8,Port_Data.Data_Transfer[189])OTL(Port_Data.Port_Read.[Port])OTL(Local_Control.4);
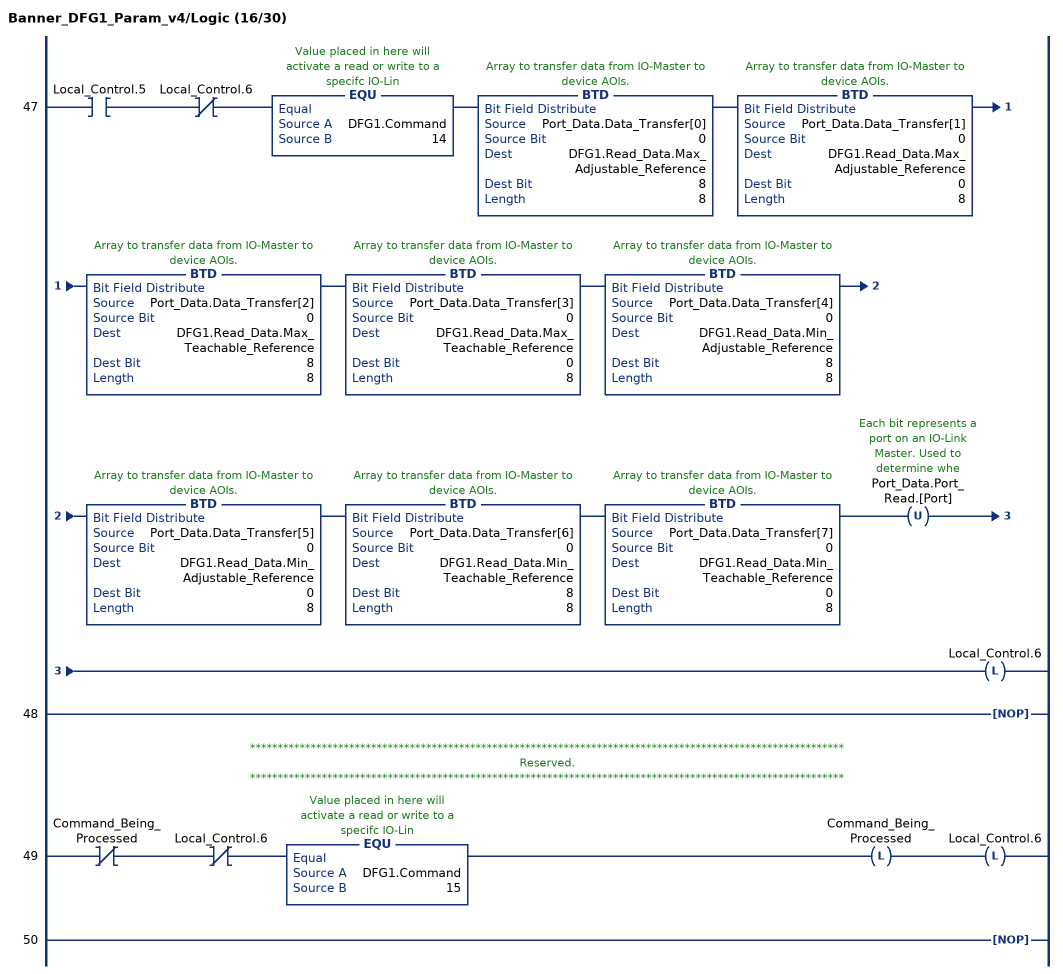
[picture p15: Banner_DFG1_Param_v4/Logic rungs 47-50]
   47: XIC(Local_Control.5)XIO(Local_Control.6)EQU(DFG1.Command,14)BTD(Port_Data.Data_Transfer[0],0,DFG1.Read_Data.Max_Adjustable_Reference,8,8)BTD(Port_Data.Data_Transfer[1],0,DFG1.Read_Data.Max_Adjustable_Reference,0,8)BTD(Port_Data.Data_Transfer[2],0,DFG1.Read_Data.Max_Teachable_Reference,8,8)BTD(Port_Data.Data_Transfer[3],0,DFG1.Read_Data.Max_Teachable_Reference,0,8)BTD(Port_Data.Data_Transfer[4],0,DFG1.Read_Data.Min_Adjustable_Reference,8,8)BTD(Port_Data.Data_Transfer[5],0,DFG1.Read_Data.Min_Adjustable_Reference,0,8)BTD(Port_Data.Data_Transfer[6],0,DFG1.Read_Data.Min_Teachable_Reference,8,8)BTD(Port_Data.Data_Transfer[7],0,DFG1.Read_Data.Min_Teachable_Reference,0,8)OTU(Port_Data.Port_Read.[Port])OTL(Local_Control.6);
   48: NOP();
   // ************************************************************************************************************
   // Reserved.
   // ************************************************************************************************************
   49: XIO(Command_Being_Processed)XIO(Local_Control.6)EQU(DFG1.Command,15)OTL(Command_Being_Processed)OTL(Local_Control.6);
   50: NOP();
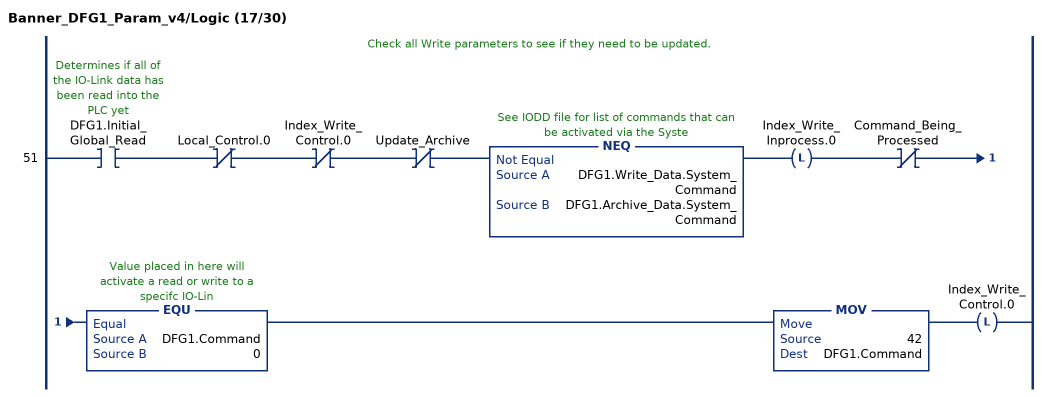
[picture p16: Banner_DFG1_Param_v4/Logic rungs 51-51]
   // Check all Write parameters to see if they need to be updated.
   51: XIC(DFG1.Initial_Global_Read)XIO(Local_Control.0)XIO(Index_Write_Control.0)XIO(Update_Archive)NEQ(DFG1.Write_Data.System_Command,DFG1.Archive_Data.System_Command)OTL(Index_Write_Inprocess.0)XIO(Command_Being_Processed)EQU(DFG1.Command,0)MOV(42,DFG1.Command)OTL(Index_Write_Control.0);
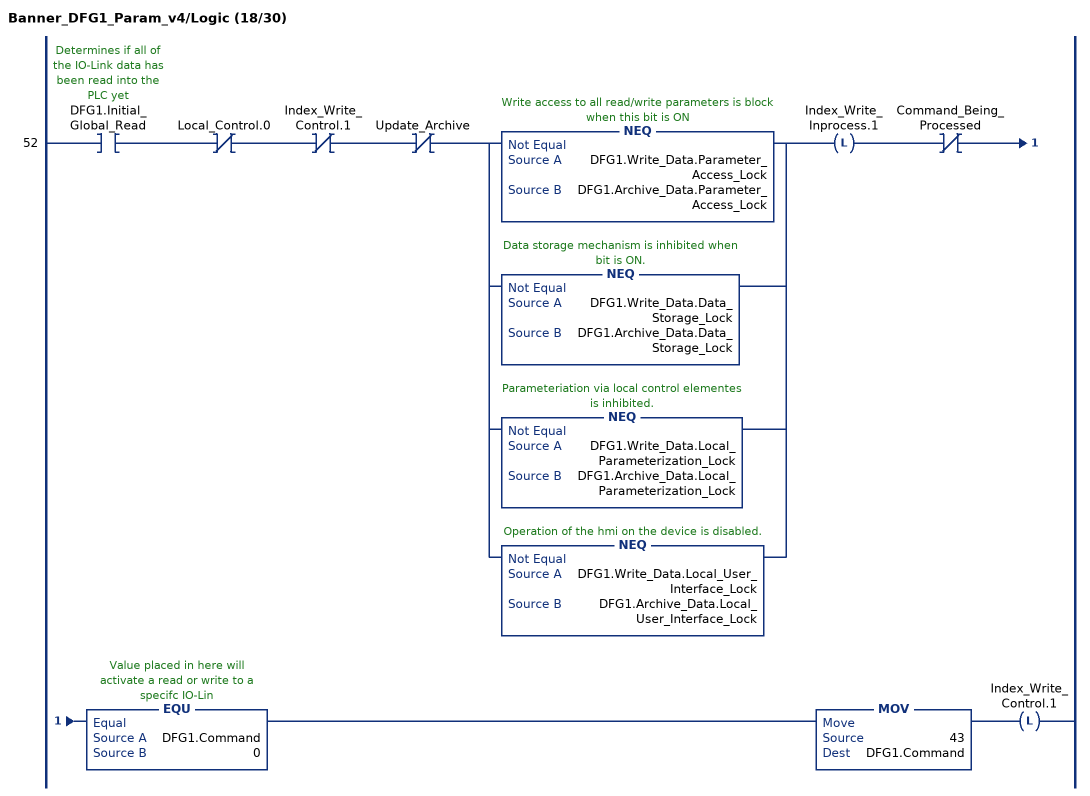
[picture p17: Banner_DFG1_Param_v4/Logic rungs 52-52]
   52: XIC(DFG1.Initial_Global_Read)XIO(Local_Control.0)XIO(Index_Write_Control.1)XIO(Update_Archive)[NEQ(DFG1.Write_Data.Parameter_Access_Lock,DFG1.Archive_Data.Parameter_Access_Lock) ,NEQ(DFG1.Write_Data.Data_Storage_Lock,DFG1.Archive_Data.Data_Storage_Lock) ,NEQ(DFG1.Write_Data.Local_Parameterization_Lock,DFG1.Archive_Data.Local_Parameterization_Lock) ,NEQ(DFG1.Write_Data.Local_User_Interface_Lock,DFG1.Archive_Data.Local_User_Interface_Lock) ]OTL(Index_Write_Inprocess.1)XIO(Command_Being_Processed)EQU(DFG1.Command,0)MOV(43,DFG1.Command)OTL(Index_Write_Control.1);
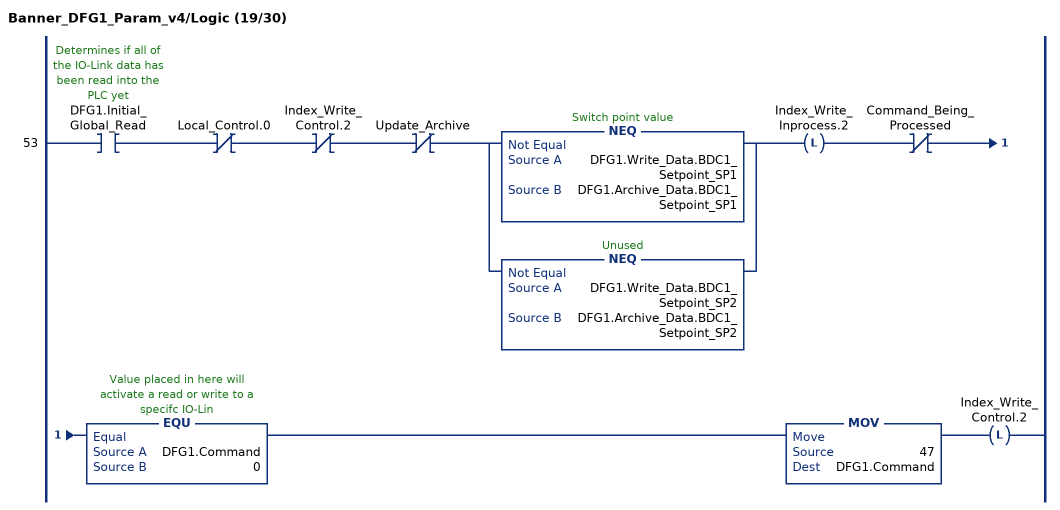
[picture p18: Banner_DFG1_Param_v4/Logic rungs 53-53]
   53: XIC(DFG1.Initial_Global_Read)XIO(Local_Control.0)XIO(Index_Write_Control.2)XIO(Update_Archive)[NEQ(DFG1.Write_Data.BDC1_Setpoint_SP1,DFG1.Archive_Data.BDC1_Setpoint_SP1) ,NEQ(DFG1.Write_Data.BDC1_Setpoint_SP2,DFG1.Archive_Data.BDC1_Setpoint_SP2) ]OTL(Index_Write_Inprocess.2)XIO(Command_Being_Processed)EQU(DFG1.Command,0)MOV(47,DFG1.Command)OTL(Index_Write_Control.2);
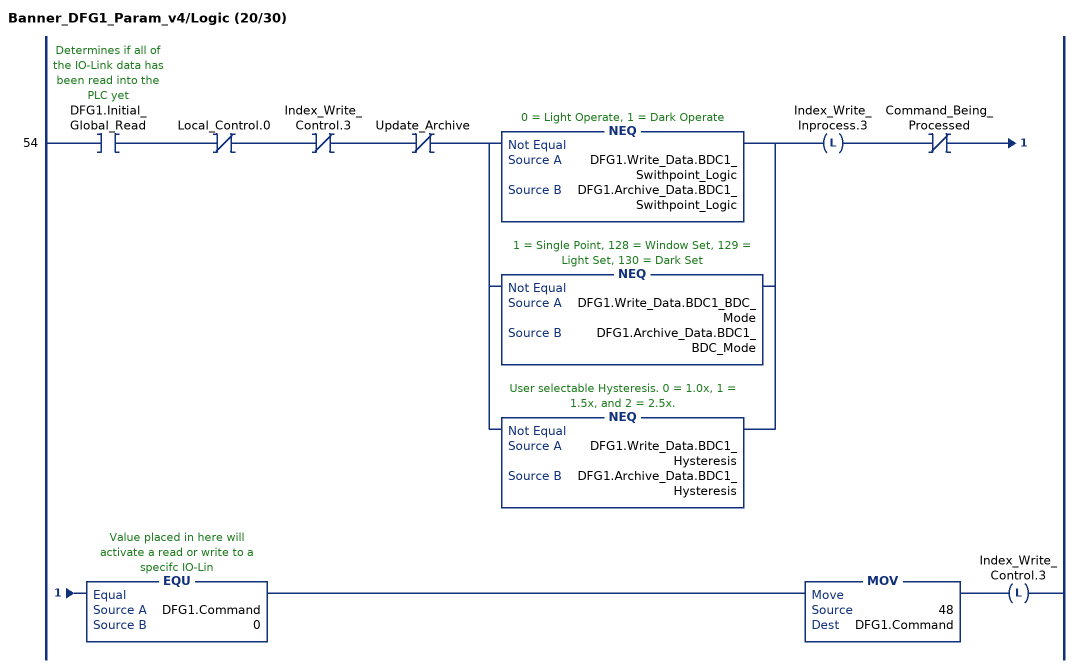
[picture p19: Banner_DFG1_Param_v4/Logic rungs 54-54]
   54: XIC(DFG1.Initial_Global_Read)XIO(Local_Control.0)XIO(Index_Write_Control.3)XIO(Update_Archive)[NEQ(DFG1.Write_Data.BDC1_Swithpoint_Logic,DFG1.Archive_Data.BDC1_Swithpoint_Logic) ,NEQ(DFG1.Write_Data.BDC1_BDC_Mode,DFG1.Archive_Data.BDC1_BDC_Mode) ,NEQ(DFG1.Write_Data.BDC1_Hysteresis,DFG1.Archive_Data.BDC1_Hysteresis) ]OTL(Index_Write_Inprocess.3)XIO(Command_Being_Processed)EQU(DFG1.Command,0)MOV(48,DFG1.Command)OTL(Index_Write_Control.3);
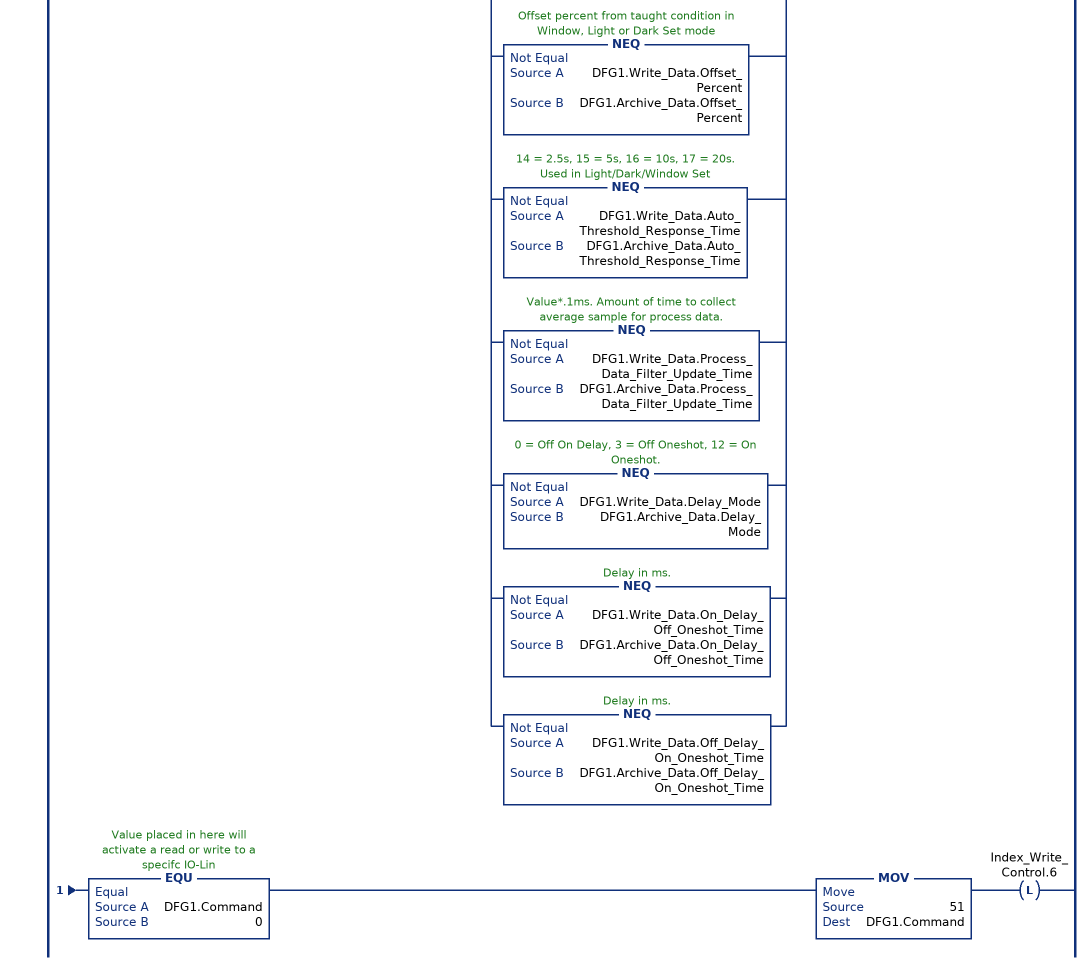
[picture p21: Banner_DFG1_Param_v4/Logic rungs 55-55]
   55: XIC(DFG1.Initial_Global_Read)XIO(Local_Control.0)XIO(Index_Write_Control.6)XIO(Update_Archive)[NEQ(DFG1.Write_Data.Signal_Theshold_Readout,DFG1.Archive_Data.Signal_Theshold_Readout) ,NEQ(DFG1.Write_Data.ECO_Mode,DFG1.Archive_Data.ECO_Mode) ,NEQ(DFG1.Write_Data.Display_Orientation,DFG1.Archive_Data.Display_Orientation) ,NEQ(DFG1.Write_Data.Gain_Level,DFG1.Archive_Data.Gain_Level) ,NEQ(DFG1.Write_Data.Gain_Mode,DFG1.Archive_Data.Gain_Mode) ,NEQ(DFG1.Write_Data.Response_Speed,DFG1.Archive_Data.Response_Speed) ,NEQ(DFG1.Write_Data.Teach_Selection,DFG1.Archive_Data.Teach_Selection) ,NEQ(DFG1.Write_Data.Auto_Treshold,DFG1.Archive_Data.Auto_Treshold) ,NEQ(DFG1.Write_Data.Offset_Percent,DFG1.Archive_Data.Offset_Percent) ,NEQ(DFG1.Write_Data.Auto_Threshold_Response_Time,DFG1.Archive_Data.Auto_Threshold_Response_Time) ,NEQ(DFG1.Write_Data.Process_Data_Filter_Update_Time,DFG1.Archive_Data.Process_Data_Filter_Update_Time) ,NEQ(DFG1.Write_Data.Delay_Mode,DFG1.Archive_Data.Delay_Mode) ,NEQ(DFG1.Write_Data.On_Delay_Off_Oneshot_Time,DFG1.Archive_Data.On_Delay_Off_Oneshot_Time) ,NEQ(DFG1.Write_Data.Off_Delay_On_Oneshot_Time,DFG1.Archive_Data.Off_Delay_On_Oneshot_Time) ]OTL(Index_Write_Inprocess.6)XIO(Command_Being_Processed)EQU(DFG1.Command,0)MOV(51,DFG1.Command)OTL(Index_Write_Control.6);
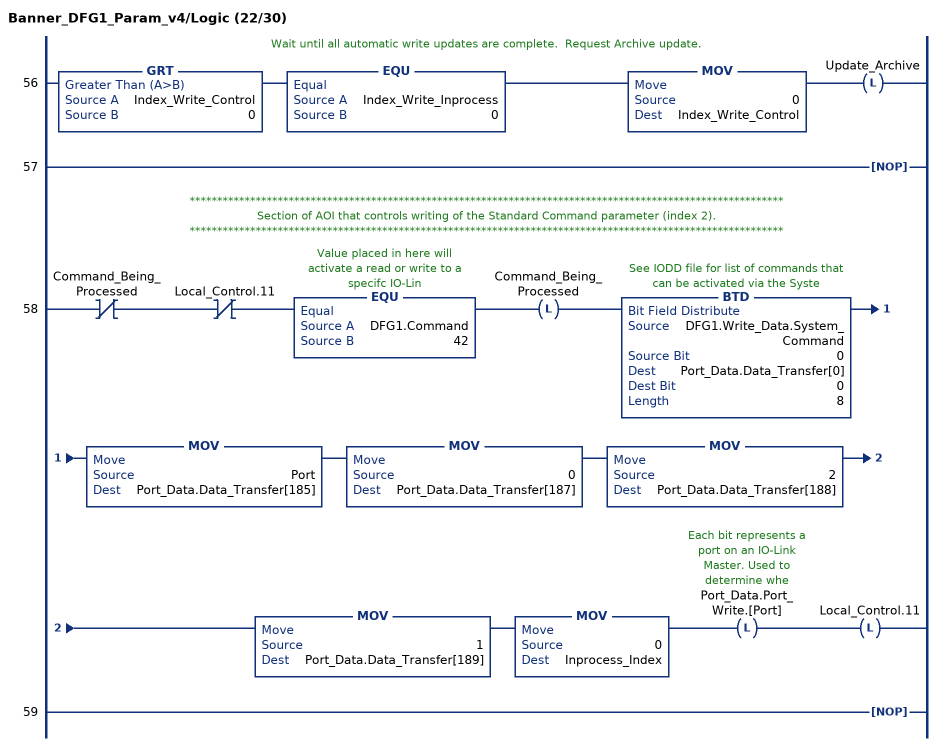
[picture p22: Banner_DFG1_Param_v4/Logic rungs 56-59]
   // Wait until all automatic write updates are complete.  Request Archive update.
   56: GRT(Index_Write_Control,0)EQU(Index_Write_Inprocess,0)MOV(0,Index_Write_Control)OTL(Update_Archive);
   57: NOP();
   // ************************************************************************************************************
   // Section of AOI that controls writing of the Standard Command parameter (index 2).
   // ************************************************************************************************************
   58: XIO(Command_Being_Processed)XIO(Local_Control.11)EQU(DFG1.Command,42)OTL(Command_Being_Processed)BTD(DFG1.Write_Data.System_Command,0,Port_Data.Data_Transfer[0],0,8)MOV(Port,Port_Data.Data_Transfer[185])MOV(0,Port_Data.Data_Transfer[187])MOV(2,Port_Data.Data_Transfer[188])MOV(1,Port_Data.Data_Transfer[189])MOV(0,Inprocess_Index)OTL(Port_Data.Port_Write.[Port])OTL(Local_Control.11);
   59: NOP();
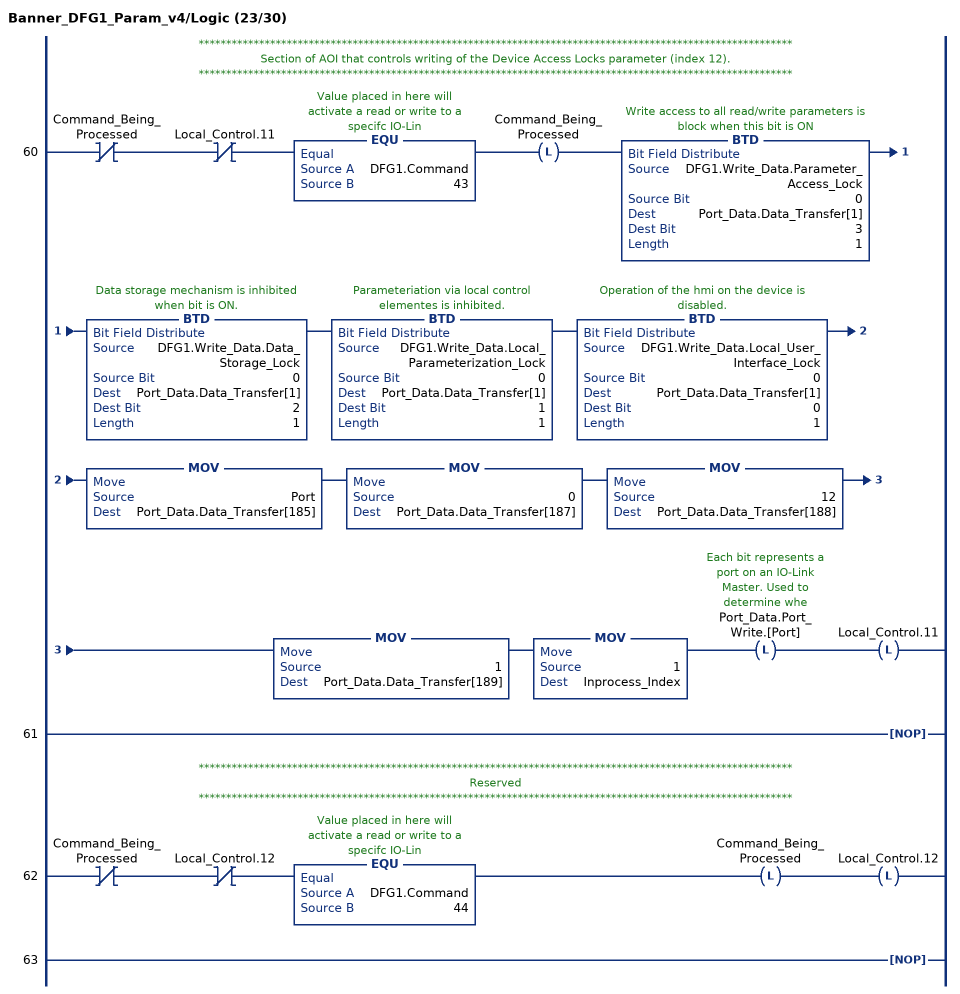
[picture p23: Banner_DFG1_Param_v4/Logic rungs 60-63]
   // ************************************************************************************************************
   // Section of AOI that controls writing of the Device Access Locks parameter (index 12).
   // ************************************************************************************************************
   60: XIO(Command_Being_Processed)XIO(Local_Control.11)EQU(DFG1.Command,43)OTL(Command_Being_Processed)BTD(DFG1.Write_Data.Parameter_Access_Lock,0,Port_Data.Data_Transfer[1],3,1)BTD(DFG1.Write_Data.Data_Storage_Lock,0,Port_Data.Data_Transfer[1],2,1)BTD(DFG1.Write_Data.Local_Parameterization_Lock,0,Port_Data.Data_Transfer[1],1,1)BTD(DFG1.Write_Data.Local_User_Interface_Lock,0,Port_Data.Data_Transfer[1],0,1)MOV(Port,Port_Data.Data_Transfer[185])MOV(0,Port_Data.Data_Transfer[187])MOV(12,Port_Data.Data_Transfer[188])MOV(1,Port_Data.Data_Transfer[189])MOV(1,Inprocess_Index)OTL(Port_Data.Port_Write.[Port])OTL(Local_Control.11);
   61: NOP();
   // ************************************************************************************************************
   // Reserved
   // ************************************************************************************************************
   62: XIO(Command_Being_Processed)XIO(Local_Control.12)EQU(DFG1.Command,44)OTL(Command_Being_Processed)OTL(Local_Control.12);
   63: NOP();
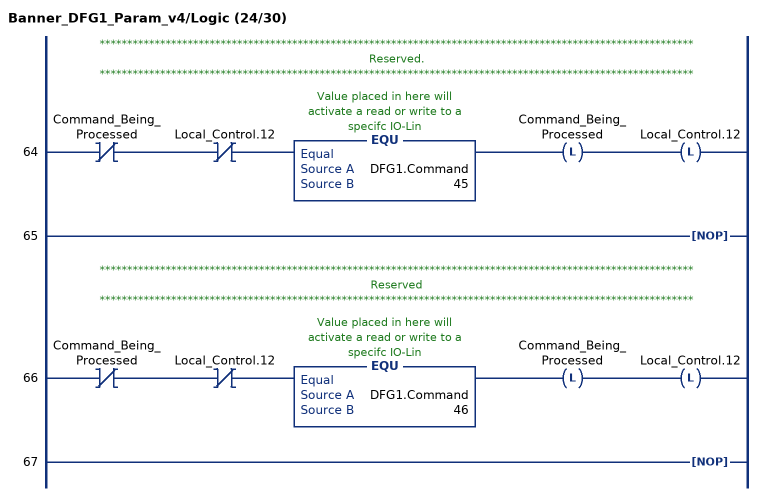
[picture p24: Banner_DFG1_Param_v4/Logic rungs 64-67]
   // ************************************************************************************************************
   // Reserved.
   // ************************************************************************************************************
   64: XIO(Command_Being_Processed)XIO(Local_Control.12)EQU(DFG1.Command,45)OTL(Command_Being_Processed)OTL(Local_Control.12);
   65: NOP();
   // ************************************************************************************************************
   // Reserved
   // ************************************************************************************************************
   66: XIO(Command_Being_Processed)XIO(Local_Control.12)EQU(DFG1.Command,46)OTL(Command_Being_Processed)OTL(Local_Control.12);
   67: NOP();
